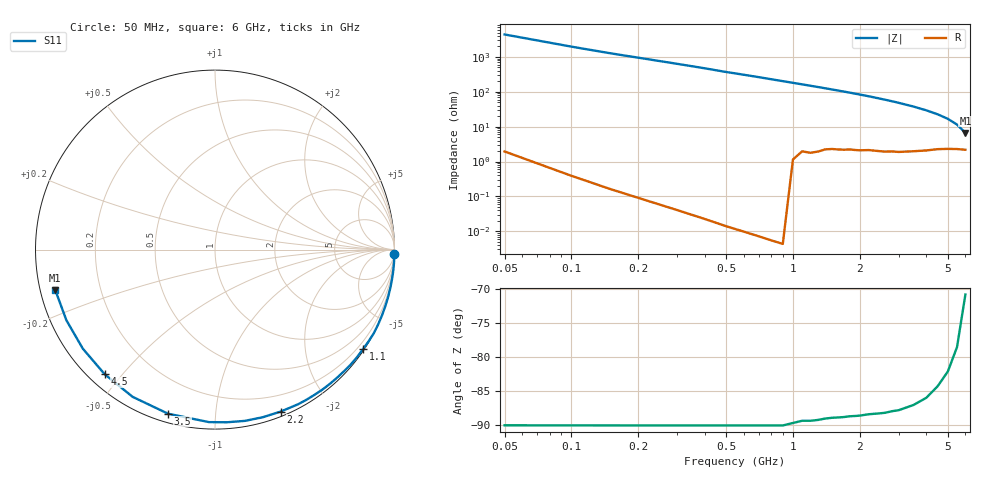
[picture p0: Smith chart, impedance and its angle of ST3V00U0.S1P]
! SIEMENS Discrete & RF Semiconductors
! BA892
! Si PIN Diode in SCD-80
! VR = 3 V
! S-Parameters:  September  1997
# GHz  S  MA  R  50
!  f  S11
! GHz  MAG  ANG
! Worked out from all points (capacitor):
!   34 points, 50 MHz to 6 GHz, reference 50 ohm
!   read as one part to ground: C = 806 fF near 50 MHz
!   lowest |Z| = 6.63 ohm at 6 GHz (marker M1)
!   S11 on the Smith chart (normalised r, x): 50 MHz: 0, -88; 1.1 GHz: 0.04, -3.27; 2.2 GHz: 0.04, -1.48; 3.5 GHz: 0.04, -0.75; 4.5 GHz: 0.05, -0.45; 6 GHz: 0.04, -0.13
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0.05  1 -1.3
0.15  1 -4.5
0.25  1 -7.5
0.4  1 -12.1
0.5  1 -15.4
0.6  1 -18.4
0.7  1 -21.5
0.8  1 -24.7
0.9  1 -27.8
1.1  0.9933 -34.0
1.2  0.9928 -37.1
1.3  0.9909 -40.2
1.5  0.9859 -46.3
1.6  0.9846 -49.5
1.7  0.9831 -52.5
1.9  0.9796 -58.7
2  0.9781 -61.8
2.2  0.9737 -67.9
2.4  0.9711 -74.1
2.6  0.9687 -80.1
2.8  0.9643 -86.1
3  0.9618 -92.0
3.5  0.9509 -106.0
4  0.94 -119.2
4.5  0.9274 -131.5
5  0.9203 -143.2
5.5  0.9167 -154.6
6  0.9178 -165.7
